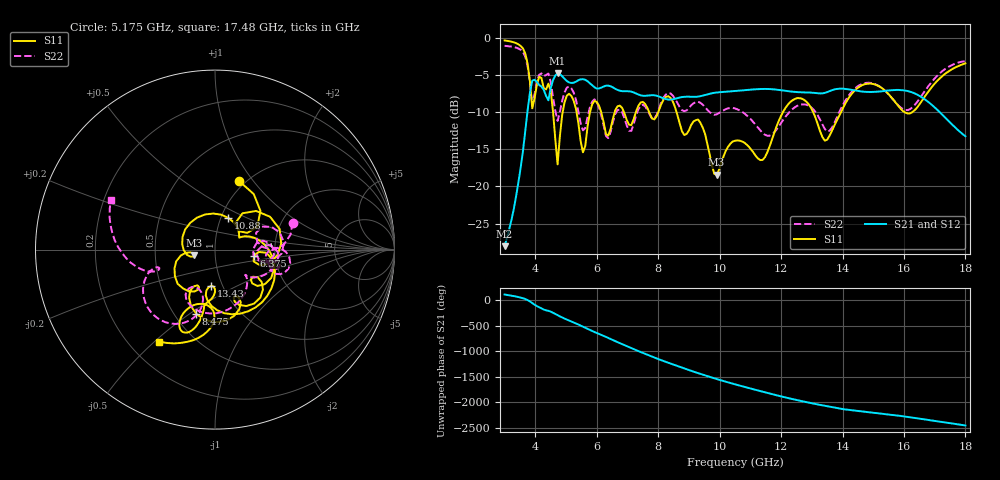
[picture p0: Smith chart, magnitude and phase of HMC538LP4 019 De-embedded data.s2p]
! Chelmsford, MA 01824
! http://www.hittite.com
! Tel: 978-250-3343
! Fax: 978-250-3373
! Device  :  HMC538LP4
! Description:  600 Analog Phase Shifter
! Frequency  :  6.0 GHz - 15.0 GHz
! Package  :  LP4  - 4x4 mm Quad Flatpack No-Lead (QFN) Plastic Package: 24 pin
! Ports  :  2 RF, 1 DC
!  Pin  3  = Rfin  = Port 1
!  Pin  16  = Rfout = Port 2
!  pin  21  = vCTL
! Voltages:  VCTL  = 0 to 5.0 Volts
! Currents :  Vb(V)  Vd(V)  Ib(mA)  Id(mA)
!  0.00  1.90  0.000000	0.477450
! Data:  The device was measured on evaluation board 111296-1.
!  Data was collected using a calibrated network analyzer.
!  The evaluation circuit board was modeled and simulated.This was use
!  to removed the evaluation board circuit from the measured data.
!  The reference plane is the center of the package pin.
! Misc:  Lot #
!Date Measured:  03 - 11 -2009
! Date:  03 - 17 -2009
! Note:
!  Hittite Microwave supplies this data as a sample of measured data at the
!  package pin for this package product.  Your particular data for this product
!  may vary.
!  Data was taken at 25 degrees C.
!  Hittite Microwave reserves the right to change this data at anytime.
# MHz S MA R 50
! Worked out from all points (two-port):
!   201 points, 3 GHz to 18 GHz, reference 50 ohm
!   highest |S21| = -4.76 dB at 4.725 GHz (marker M1); lowest = -28.0 dB at 3 GHz (marker M2)
!   |S21| within 3 dB of the highest: 4.454 GHz to 7.474 GHz (3.02 GHz wide, 50.6 % of centre); 9.456 GHz to 16.49 GHz (7.034 GHz wide, 54.2 % of centre)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
!   lowest |S11| = -18.4 dB at 9.9 GHz (marker M3), VSWR 1.27, Z = 39.6 - j2.6 ohm
!   |S11| at or under -10 dB: 5.343 GHz to 5.779 GHz (436.4 MHz wide, 7.85 % of centre); 8.598 GHz to 12.06 GHz (3.462 GHz wide, 33.5 % of centre); 13.05 GHz to 13.95 GHz (906.4 MHz wide, 6.72 % of centre)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
!   |S22| runs from -13.5 to -1.1 dB; largest |S21 - S12| = 0.0033
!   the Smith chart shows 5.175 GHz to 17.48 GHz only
!   S11 on the Smith chart (normalised r, x): 5.175 GHz: 0.93, +0.85; 6.375 GHz: 1.55, -0.11; 8.475 GHz: 0.64, -0.53; 10.88 GHz: 1.08, +0.40; 13.43 GHz: 0.88, -0.37; 17.48 GHz: 0.32, -0.52
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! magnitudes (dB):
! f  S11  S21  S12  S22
! 3 GHz  -0.3  -28.0  -28.0  -1.1
! 3.675 GHz  -2.1  -12.4  -12.4  -2.5
! 3.9 GHz  -9.5  -5.7  -5.7  -9.1
! 4.425 GHz  -6.1  -8.4  -8.4  -4.8
! 4.725 GHz  -17.0  -4.8  -4.8  -11.2
! 4.95 GHz  -8.7  -5.5  -5.5  -7.3
! 5.175 GHz  -7.8  -6.1  -6.1  -6.8
! 5.55 GHz  -15.4  -5.6  -5.6  -12.4
! 5.925 GHz  -8.5  -6.6  -6.6  -8.3
! 6.375 GHz  -13.1  -6.4  -6.4  -13.5
! 8.025 GHz  -9.7  -7.9  -7.9  -9.5
! 8.475 GHz  -8.6  -8.3  -8.3  -7.8
! 9.9 GHz  -18.4  -7.3  -7.4  -10.3
! 10.5 GHz  -13.8  -7.2  -7.2  -9.5
! 10.88 GHz  -14.3  -7.0  -7.0  -10.4
! 13.05 GHz  -10.0  -7.4  -7.4  -9.6
! 13.43 GHz  -13.8  -7.4  -7.4  -12.3
! 14.55 GHz  -6.6  -7.2  -7.2  -6.4
! 15.53 GHz  -7.7  -7.1  -7.1  -7.7
! 16.2 GHz  -10.2  -7.2  -7.3  -9.6
! 17.48 GHz  -4.4  -11.3  -11.3  -3.8
! 18 GHz  -3.4  -13.2  -13.2  -3.1
